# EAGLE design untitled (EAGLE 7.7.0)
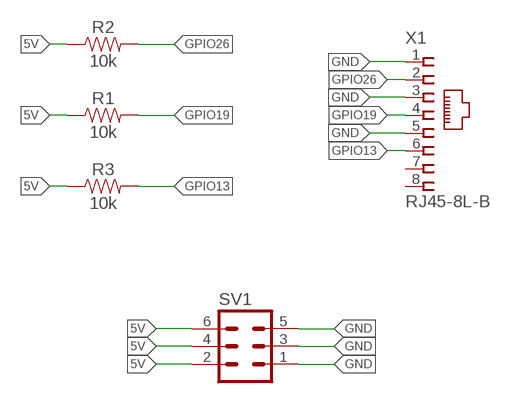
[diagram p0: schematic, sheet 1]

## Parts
R1  10k  10KOHM-HORIZ-1/4W-1%  [AXIAL-0.3]
R2  10k  10KOHM-HORIZ-1/4W-1%  [AXIAL-0.3]
R3  10k  10KOHM-HORIZ-1/4W-1%  [AXIAL-0.3]
SV1  MA03-2  [MA03-2]
X1  RJ45-8L-B  [RJ45-NO-SHIELD]

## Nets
5V: R1.P$1 R2.P$1 R3.P$1 SV1.2 SV1.4 SV1.6
GND: SV1.1 SV1.3 SV1.5 X1.1 X1.3 X1.5
GPIO13: R3.P$2 X1.6
GPIO19: R1.P$2 X1.4
GPIO26: R2.P$2 X1.2
Unconnected: X1.7 X1.8

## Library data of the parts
R1-R3 = SparkFun-Resistors:10KOHM: 10kΩ resistor; PROD_ID: RES-12183
SV1 = con-lstb:MA03-2: PIN HEADER; OC_FARNELL: unknown; OC_NEWARK: unknown
X1 = con-tycoelectronics:RJ45: CORCOM Modular RJ Jacks No Shield Source: www.tycoelectronics.com .. ENG_DS_1654001_1099_RJ_L_0507.pdf; MF: TYCO ELECTRONICS; MPN: RJ45-8L-B; OC_FARNELL: 1279843; OC_NEWARK: 52K4445

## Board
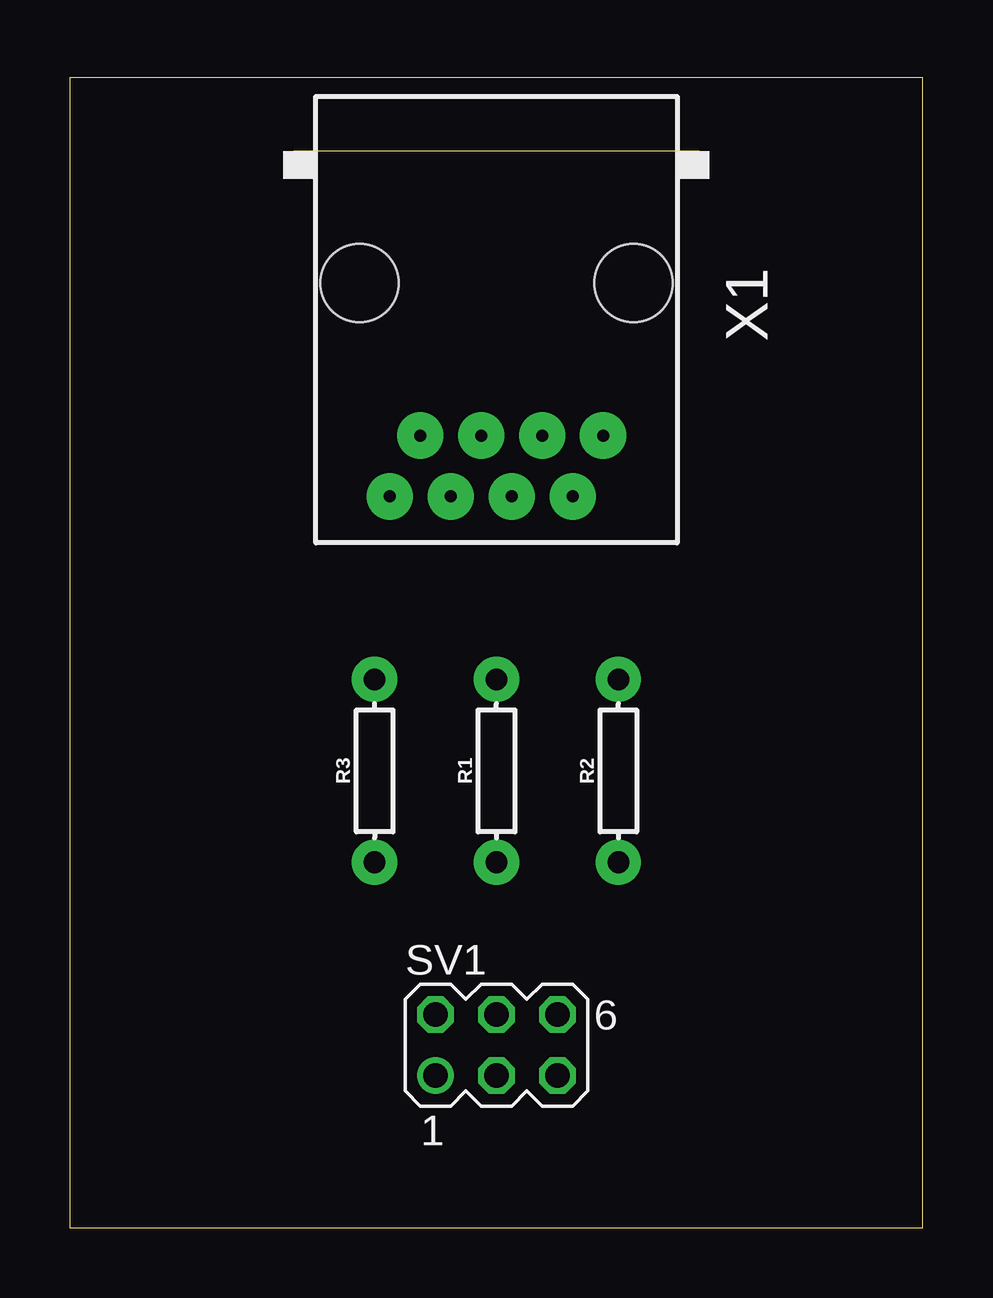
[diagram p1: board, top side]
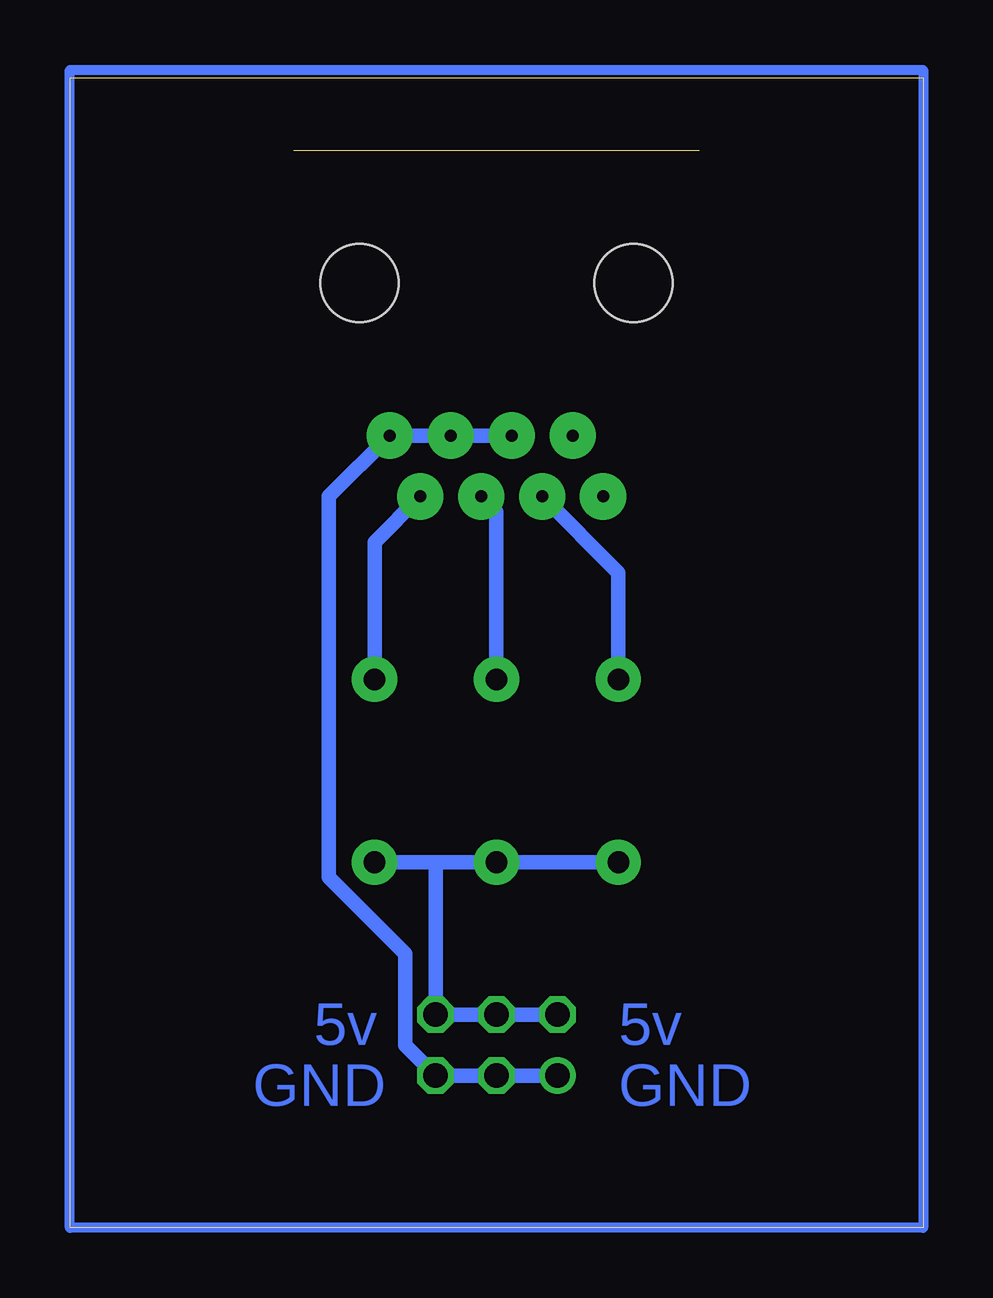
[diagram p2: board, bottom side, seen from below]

Size 35.54 x 47.93 mm. Coordinates in mm from the lower left corner, seen from the top.
Outline: 0,0 35.54,0 35.54,47.93 0,47.93 0,0
Copper layers (1*16): Top 0.035mm / dielectric 1.5mm / Bottom 0.035mm
Design rules "default *": minimum track width 24mil, minimum drill 24mil, track to track 8mil, track to pad 8mil, pad to pad 8mil, via to via 8mil, smd to smd 8mil, copper to edge 40mil, drill to drill 8mil, minimum pad ring 10mil, minimum via ring 8mil, stop-mask expansion 4mil, vias tented up to drill 0mil, thermal gap 10mil

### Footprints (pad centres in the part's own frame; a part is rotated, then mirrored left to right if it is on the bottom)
AXIAL-0.3 = drill 0.9 pad 1.88: P$1 -3.81,0; P$2 3.81,0
MA03-2 = drill 1.016: 1 -2.54,-1.27 | drill 1.016 octagon: 2 -2.54,1.27; 3 0,-1.27; 4 0,1.27; 5 2.54,-1.27; 6 2.54,1.27
RJ45-NO-SHIELD = drill 0.5 pad 1.93: 1 -4.445,6.35; 2 -3.175,8.89; 3 -1.905,6.35; 4 -0.635,8.89; 5 0.635,6.35; 6 1.905,8.89; 7 3.175,6.35; 8 4.445,8.89 | hole 3.251: -5.715,0; 5.715,0

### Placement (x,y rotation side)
R1  17.78,19.05 90 top
R2  22.86,19.05 90 top
R3  12.7,19.05 90 top
SV1  17.78,7.62 0 top
X1  17.78,39.37 180 top

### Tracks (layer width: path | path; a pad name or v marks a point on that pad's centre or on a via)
5V
  Bottom 0.61: SV1.2 SV1.4 SV1.6 20.32,15.24 | R3.P$1 R1.P$1 20.32,15.24 | 20.32,15.24 R2.P$1
GND
  Bottom 0.61: SV1.1 SV1.3 SV1.5 21.59,7.62 21.59,11.43 24.77,14.6 24.77,30.48 X1.1 X1.3 X1.5
GPIO13
  Bottom 0.61: R3.P$2 12.7,27.3 X1.6
GPIO19
  Bottom 0.61: R1.P$2 17.78,29.84 X1.4
GPIO26
  Bottom 0.61: R2.P$2 22.86,28.58 X1.2
N$1
  Bottom 0.406: 0,48.26 0,0 35.56,0 35.56,48.26 0,48.26

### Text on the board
Bottom: 5v | 5v | GND | GND

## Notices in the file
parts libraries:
SparkFun-Resistors: Licensing: Creative Commons ShareAlike 4.0 International - https://creativecommons.org/licenses/by-sa/4.0
